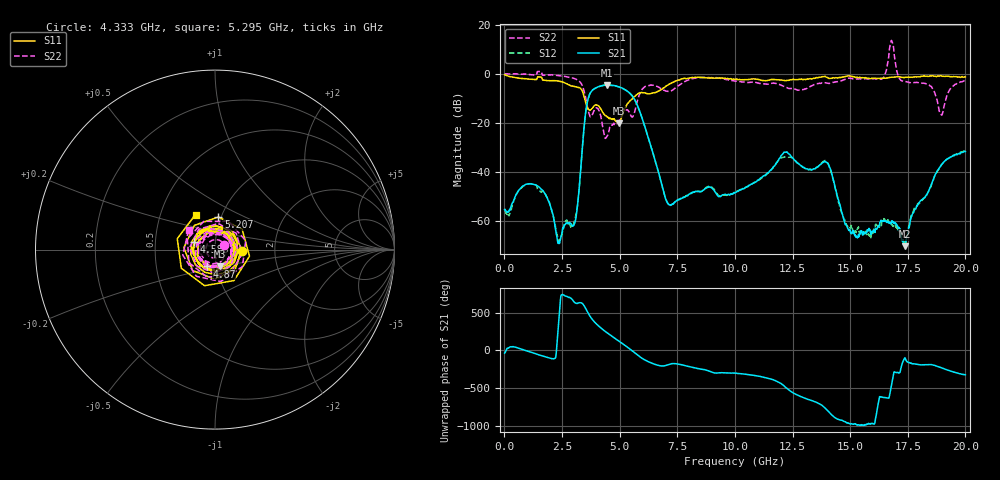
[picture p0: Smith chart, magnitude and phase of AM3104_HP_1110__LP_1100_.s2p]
!Created with skrf (http://scikit-rf.org).
# Hz S RI R 50.0
!freq ReS11 ImS11 ReS21 ImS21 ReS12 ImS12 ReS22 ImS22
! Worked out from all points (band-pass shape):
!   1601 points, 10 MHz to 20 GHz, reference 50 ohm
!   highest |S21| = -4.61 dB at 4.458 GHz (marker M1); lowest = -70.3 dB at 17.38 GHz (marker M2)
!   |S21| within 3 dB of the highest: 3.743 GHz to 5.395 GHz (1.653 GHz wide, 36.2 % of centre)
!   lowest |S11| = -20.2 dB at 4.958 GHz (marker M3), VSWR 1.22, Z = 52 - j9.78 ohm
!   |S11| at or under -10 dB: 3.475 GHz to 5.576 GHz (2.102 GHz wide, 46.4 % of centre)
!   |S22| runs from -26.4 to 13.5 dB; largest |S21 - S12| = 0.057
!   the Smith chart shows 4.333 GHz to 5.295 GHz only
!   S11 on the Smith chart (normalised r, x): 4.333 GHz: 1.35, -0.03; 4.583 GHz: 0.79, +0.07; 4.87 GHz: 0.90, -0.17; 5.207 GHz: 0.97, +0.36; 5.295 GHz: 0.75, +0.31
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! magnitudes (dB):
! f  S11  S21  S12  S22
! 10 MHz  -0.4  -55.4  -55.5  -0.1
! 1.422 GHz  -1.9  -45.6  -46.5  0.5
! 2.384 GHz  -3.1  -68.9  -68.5  -0.8
! 3.058 GHz  -5.3  -60.9  -59.7  -2.1
! 3.346 GHz  -6.5  -34.8  -34.9  -4.2
! 3.658 GHz  -14.7  -9.5  -9.6  -15.9
! 4.333 GHz  -16.6  -4.7  -4.7  -24.8
! 4.458 GHz  -17.6  -4.6  -4.6  -25.5
! 4.583 GHz  -18.1  -4.7  -4.8  -21.6
! 4.87 GHz  -19.6  -5.1  -5.1  -20.5
! 4.958 GHz  -20.2  -5.3  -5.4  -19.7
! 5.207 GHz  -14.8  -6.4  -6.4  -15.4
! 5.295 GHz  -13.0  -6.9  -6.9  -14.8
! 6.682 GHz  -7.2  -40.0  -40.1  -5.4
! 7.169 GHz  -4.2  -53.5  -53.3  -7.2
! 10.01 GHz  -2.4  -48.6  -48.4  -3.1
! 13.34 GHz  -2.1  -39.2  -39.1  -4.9
! 15.25 GHz  -1.5  -66.7  -64.9  -2.2
! 16.68 GHz  -1.6  -60.4  -60.4  7.2
! 17.38 GHz  -1.5  -70.3  -69.2  -3.2
! 18.95 GHz  -0.9  -37.3  -37.4  -16.7
! 20 GHz  -1.3  -31.8  -31.2  -2.9
